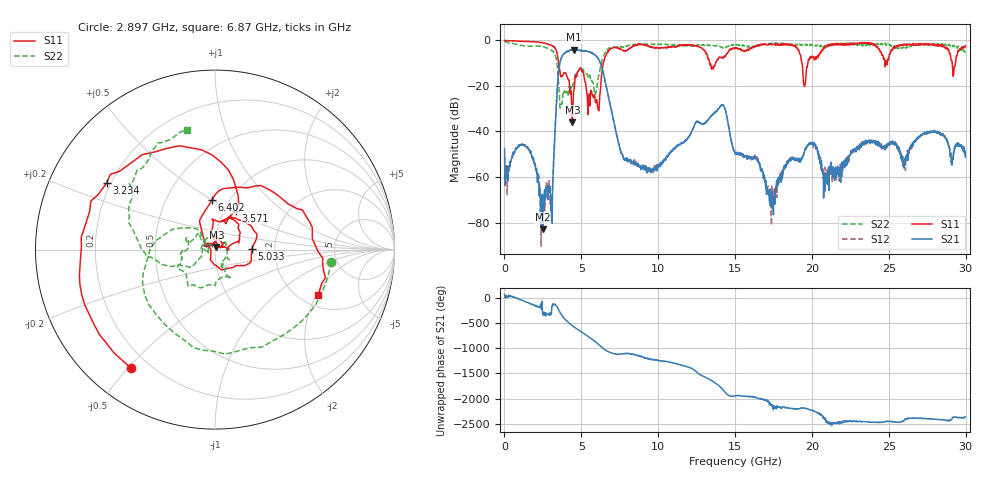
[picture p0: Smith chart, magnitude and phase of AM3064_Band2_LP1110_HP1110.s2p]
# Hz S DB R 50.0
!freq dBS11 angS11 dBS21 angS21 dBS12 angS12 dBS22 angS22
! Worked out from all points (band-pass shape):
!   1600 points, 10 MHz to 29.98 GHz, reference 50 ohm
!   highest |S21| = -4.11 dB at 4.508 GHz (marker M1); lowest = -83.0 dB at 2.484 GHz (marker M2)
!   |S21| within 3 dB of the highest: 3.743 GHz to 6 GHz (2.258 GHz wide, 46.3 % of centre)
!   lowest |S11| = -36.0 dB at 4.415 GHz (marker M3), VSWR 1.03, Z = 50.7 + j1.42 ohm
!   |S11| at or under -10 dB: 3.519 GHz to 6.429 GHz (2.91 GHz wide, 58.5 % of centre); 13.34 GHz to 13.73 GHz (395.1 MHz wide, 2.92 % of centre); 19.36 GHz to 19.73 GHz (378.2 MHz wide, 1.94 % of centre)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
!   |S22| runs from -29.7 to -0.3 dB; largest |S21 - S12| = 0.016
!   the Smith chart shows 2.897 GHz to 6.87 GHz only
!   S11 on the Smith chart (normalised r, x): 2.897 GHz: 0.13, -0.51; 3.234 GHz: 0.18, +0.27; 3.571 GHz: 1.14, +0.53; 5.033 GHz: 1.52, +0.01; 6.402 GHz: 0.83, +0.49; 6.87 GHz: 2.50, -2.07
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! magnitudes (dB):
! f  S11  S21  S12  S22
! 10 MHz  0.0  -47.5  -51.3  -0.3
! 1.491 GHz  -0.5  -47.2  -46.8  -2.6
! 2.484 GHz  -1.0  -83.0  -69.1  -3.0
! 2.897 GHz  -1.8  -65.2  -65.3  -3.8
! 3.234 GHz  -3.0  -47.9  -48.3  -5.7
! 3.571 GHz  -12.2  -11.2  -11.1  -23.8
! 4.415 GHz  -36.0  -4.1  -4.1  -20.9
! 4.508 GHz  -22.1  -4.1  -4.1  -18.5
! 5.015 GHz  -13.3  -4.6  -4.5  -13.5
! 5.033 GHz  -13.7  -4.4  -4.4  -13.5
! 6.045 GHz  -28.8  -7.5  -7.4  -18.9
! 6.402 GHz  -11.2  -13.5  -13.5  -7.8
! 6.87 GHz  -4.0  -28.3  -28.3  -3.3
! 7.789 GHz  -4.6  -52.1  -51.3  -3.0
! 10 GHz  -3.4  -54.7  -55.4  -1.8
! 14.14 GHz  -7.4  -28.4  -28.3  -2.9
! 15 GHz  -3.3  -49.7  -49.6  -2.0
! 17.44 GHz  -1.8  -71.9  -66.0  -1.5
! 19.99 GHz  -7.0  -45.6  -45.1  -1.7
! 20.91 GHz  -2.4  -60.2  -58.5  -2.5
! 25 GHz  -8.0  -46.1  -45.2  -1.6
! 29.98 GHz  -2.4  -51.3  -49.0  -4.5
